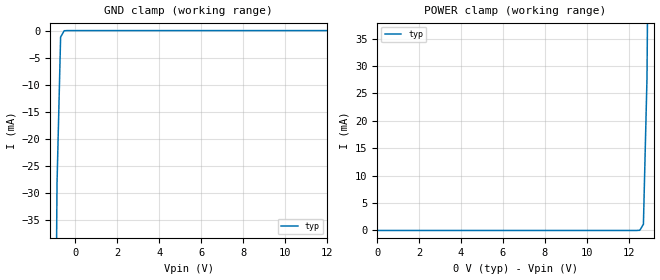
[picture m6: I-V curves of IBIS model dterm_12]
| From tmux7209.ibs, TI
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| dterm_12
[Model]   dterm_12
Model_type   Terminator
|   typ   min   max
C_comp   2.533030e-11   NA   NA
[Voltage Range]   12   0   12
[Temperature Range]   27   NA   NA
[Power Clamp Reference]   0   NA   NA
[GND Clamp Reference]   0   NA   NA
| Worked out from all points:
|   GND clamp passes 1 mA (typ) near -0.68 V on its own axis
[GND Clamp]
|   Voltage   I(typ)   I(min)   I(max)
-5V       -4.58A     NA         NA
-1.051V   -117.3mA   NA         NA
-878.8mV  -28.39mA   NA         NA
-707.1mV  -1.196mA   NA         NA
-535.4mV  -28.82uA   NA         NA
12V       1.03nA     NA         NA
[POWER Clamp]
|   Voltage   I(typ)   I(min)   I(max)
0V        -887.6pA   NA         NA
12.54V    36.36uA    NA         NA
12.71V    1.141mA    NA         NA
12.88V    28.03mA    NA         NA
13.05V    112.3mA    NA         NA
17V       5.389A     NA         NA
